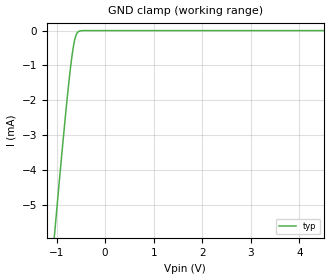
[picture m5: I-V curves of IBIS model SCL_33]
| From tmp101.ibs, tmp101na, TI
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|   SCL 3.3V Model
[Model]   SCL_33
Model_type   Input
Vinl = 0.66
Vinh = 2.31
|   typ   min   max
C_comp   4.034pF   NA   NA
[Voltage Range]   3.3   NA   NA
[Temperature Range]   27   NA   NA
[Power Clamp Reference]   3.3   NA   NA
[GND Clamp Reference]   0   NA   NA
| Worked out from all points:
|   GND clamp passes 1 mA (typ) near -0.71 V on its own axis
[GND Clamp]
|   Voltage   I(typ)   I(min)   I(max)
-3.3V     -43.26mA   NA         NA
-1.087V   -6.554mA   NA         NA
-1.014V   -5.404mA   NA         NA
-897.1mV  -3.607mA   NA         NA
-815.6mV  -2.41mA    NA         NA
-757mV    -1.606mA   NA         NA
-694.2mV  -843.1uA   NA         NA
-650.4mV  -426.3uA   NA         NA
-616.5mV  -203.9uA   NA         NA
-585.6mV  -87.78uA   NA         NA
-537.9mV  -19.8uA    NA         NA
6.59V     0A         NA         NA
[POWER Clamp]
|   SCR cell for ESD function. Effects occurr above VDD x 2
|   Voltage   I(typ)   I(min)   I(max)
-3.3V     0A         NA         NA
0V        0A         NA         NA
6.6V      0A         NA         NA
